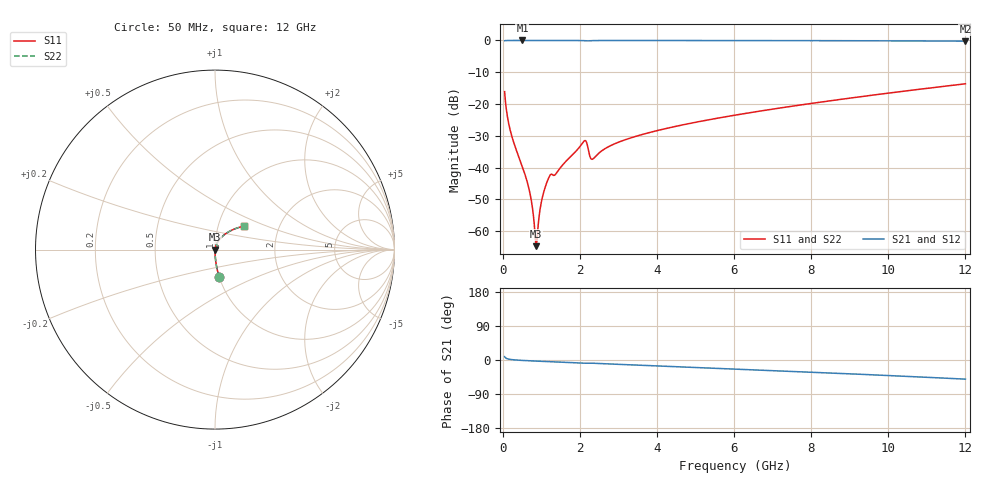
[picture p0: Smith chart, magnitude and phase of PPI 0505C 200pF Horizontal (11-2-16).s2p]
# MHz S MA R 50
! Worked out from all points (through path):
!   1601 points, 50 MHz to 12 GHz, reference 50 ohm
!   highest |S21| = 0.00 dB at 513.1 MHz (marker M1); lowest = -0.2 dB at 12 GHz (marker M2)
!   group delay of S21, straight-line fit = 11.8 ps
!   lowest |S11| = -64.7 dB at 871.6 MHz (marker M3), VSWR 1.00, Z = 50.1 - j0.000294 ohm
!   |S11| at or under -10 dB: start of sweep to end of sweep
!   |S22| runs from -64.7 to -13.6 dB; largest |S21 - S12| = 0
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50  0.1564 -81.1  0.9875 8.8  0.9875 8.8  0.1564 -81.1
214.3125  0.03486 -88.2  0.999 1.3  0.999 1.3  0.03486 -88.2
513.0625  0.01023 -88.6  0.9995 -1.1  0.9995 -1.1  0.01023 -88.6
699.7812  0.004144 -85.0  0.9994 -2.1  0.9994 -2.1  0.004144 -85.0
759.5312  0.002625 -80.6  0.9994 -2.4  0.9994 -2.4  0.002625 -80.6
834.2188  0.0009823 -57.8  0.9994 -2.7  0.9994 -2.7  0.0009823 -57.8
871.5625  0.0005797 -0.3  0.9994 -2.9  0.9994 -2.9  0.0005797 -0.3
908.9062  0.001025 51.2  0.9993 -3.1  0.9993 -3.1  0.001025 51.2
976.125  0.002328 70.6  0.9993 -3.4  0.9993 -3.4  0.002328 70.6
1028.406  0.003381 74.5  0.9992 -3.6  0.9992 -3.6  0.003381 74.5
1192.719  0.006879 73.7  0.9985 -4.4  0.9985 -4.4  0.006879 73.7
1379.438  0.007958 72.6  0.9982 -5.1  0.9982 -5.1  0.007958 72.6
2044.156  0.02314 70.1  0.9949 -8.1  0.9949 -8.1  0.02314 70.1
2148.719  0.02645 50.2  0.9858 -8.5  0.9858 -8.5  0.02645 50.2
2275.688  0.01425 42.6  0.9908 -8.2  0.9908 -8.2  0.01425 42.6
2335.438  0.0136 57.5  0.9942 -8.5  0.9942 -8.5  0.0136 57.5
2910.531  0.02375 75.5  0.9981 -11.1  0.9981 -11.1  0.02375 75.5
4038.312  0.03856 72.5  0.9977 -15.6  0.9977 -15.6  0.03856 72.5
6025  0.06677 65.1  0.996 -23.7  0.996 -23.7  0.06677 65.1
8019.156  0.1024 56.9  0.9926 -32.1  0.9926 -32.1  0.1024 56.9
10013.31  0.1486 48.2  0.9864 -41.0  0.9864 -41.0  0.1486 48.2
12000  0.2078 38.9  0.9752 -50.5  0.9752 -50.5  0.2078 38.9
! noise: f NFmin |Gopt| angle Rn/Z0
50  0.0003254  0.84  0.3054  0.0004309
1372  0.004963  0.7297  4.559  0.00365
2701  0.00689  0.6379  8.88  0.003568
4031  0.007371  0.5304  12.93  0.002734
5360  0.008888  0.4968  16.9  0.002985
6682  0.01045  0.4777  20.73  0.003309
8012  0.01206  0.4666  24.43  0.00367
9341  0.01372  0.4615  27.99  0.004069
1.067e+04  0.01545  0.4612  31.42  0.004518
1.2e+04  0.01729  0.4652  34.72  0.005031
